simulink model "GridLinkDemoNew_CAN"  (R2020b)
settings: Solver=FixedStepDiscrete  StartTime=0.0  StopTime=inf  RelTol=1e-3  EnableMultiTasking=on
InitFcn:
  | INNER_PWM=1000
  | OUTER_PWM=50000
undefined symbols (not defined in the file): A, ADCIN0, ADCIN1, ADCINA0, ADCINB0, bit, Compare, conversion, CounterCut_Outer, DCAEVT1, DCAEVT1FILT, Digital, Down, ended, Event, Filtered, GPTRIP1SEL, GPTRIP2SEL, hex2dec, identifier, input, Module, Newinv, of, Single, SPS_EMT_TAPAS_2018b, Standard, start, Tmod1, Trip, TZ1, TZ2, U_dc, Up, version, Zone
libraries: tiiqmathlib x63, c2802xlib x31, c2837xDlib x5, c280xlib x5, c28xdmclib x2, simulink x2, svdutilitieslib x1, c2000lib x1, canmsglib x1
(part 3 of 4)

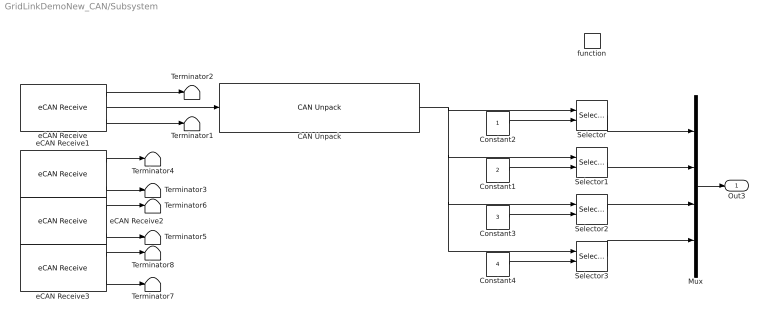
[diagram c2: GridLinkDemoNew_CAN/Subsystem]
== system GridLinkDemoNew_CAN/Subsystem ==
  function : TriggerPort  TriggerType=function-call  VariantControl=Variant
  CAN Unpack : canmsglib/CAN Unpack  MsgList=(none)  MsgName=CAN Msg  MsgIDType=Standard (11-bit identifier)  MsgIdentifier=hex2dec('01A')  MsgLength=4  SignalInfo={}  IDPort=off  TimestampPort=off  ErrorPort=off  RemotePort=off  LengthPort=off  StatusPort=off  ApplyMinMax=off
  Constant1 : Constant  Value=2  OutDataTypeStr=Inherit: Inherit via back propagation
  Constant2 : Constant  OutDataTypeStr=Inherit: Inherit via back propagation
  Constant3 : Constant  Value=3  OutDataTypeStr=Inherit: Inherit via back propagation
  Constant4 : Constant  Value=4  OutDataTypeStr=Inherit: Inherit via back propagation
  Mux : Mux
  Selector{,1..3} (4 alike) : Selector  InputPortWidth=4  IndexOptions=Index vector (port)  Indices=1  OutputSizes=1
  Terminator{1..8} (8 alike) : Terminator
  eCAN Receive : c280xlib/eCAN Receive  chipFamily=C280x  useModule=eCAN_B  mailboxNo=2  messageID=hex2dec('01A')  messageType=Standard (11-bit identifier)  sampleTime=-1  dataType=CAN_MESSAGE_TYPE  initValue=0  outputMessageLength=on  outputMessageTimeStamp=off  postInterrupt=on  interruptLine=0
  eCAN Receive1 : c280xlib/eCAN Receive  Commented=on  chipFamily=C280x  useModule=eCAN_B  mailboxNo=3  messageID=hex2dec('02A')  messageType=Standard (11-bit identifier)  sampleTime=-1  dataType=uint16  initValue=0  outputMessageLength=on  outputMessageTimeStamp=off  postInterrupt=on  interruptLine=0
  eCAN Receive2 : c280xlib/eCAN Receive  Commented=on  chipFamily=C280x  useModule=eCAN_B  mailboxNo=4  messageID=hex2dec('03A')  messageType=Standard (11-bit identifier)  sampleTime=-1  dataType=uint16  initValue=0  outputMessageLength=on  outputMessageTimeStamp=off  postInterrupt=on  interruptLine=0
  eCAN Receive3 : c280xlib/eCAN Receive  Commented=on  chipFamily=C280x  useModule=eCAN_B  mailboxNo=5  messageID=hex2dec('04A')  messageType=Standard (11-bit identifier)  sampleTime=-1  dataType=uint16  initValue=0  outputMessageLength=on  outputMessageTimeStamp=off  postInterrupt=on  interruptLine=0
  Out3 : Outport  VectorParamsAs1DForOutWhenUnconnected=off
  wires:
  eCAN Receive/1 -> Terminator2/1
  Constant2/1 -> Selector/2
  eCAN Receive/3 -> Terminator1/1
  eCAN Receive1/3 -> Terminator3/1
  Constant1/1 -> Selector1/2
  Selector1/1 -> Mux/2
  eCAN Receive1/1 -> Terminator4/1
  Constant3/1 -> Selector2/2
  eCAN Receive2/3 -> Terminator5/1
  Selector2/1 -> Mux/3
  eCAN Receive2/1 -> Terminator6/1
  Constant4/1 -> Selector3/2
  eCAN Receive3/3 -> Terminator7/1
  Selector3/1 -> Mux/4
  eCAN Receive3/1 -> Terminator8/1
  Mux/1 -> Out3/1
  Selector/1 -> Mux/1
  CAN Unpack/1 -> Selector3/1, Selector2/1, Selector1/1, Selector/1
  eCAN Receive/2 -> CAN Unpack/1

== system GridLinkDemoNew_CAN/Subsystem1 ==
  ePWM : c2802xlib/ePWM  PwmType=C2000_Type4  useModule=ePWM8  ePWMxLINKTBPRD=Not Linked  periodUnits=Clock cycles  timerSource=Specify via dialog  timerPeriod_clk=250  timerPeriod_sec=0.0001  tbshadow=Counter equals to zero  countingMode=Up-Down  phaseActiveEnable=Disable  phaseDirection=Count down after sync  phaseActive=0  synchronizationEnable=off  dcaevt1Sync=off  dcbevt1Sync=off  synchronizationOption=Disable  perSynchronizationOption=Counter equals to period (CTR=PRD)  clockPrescale=1  HSclockPrescale=1  enswap=off  ePWMxAStatus=on  ePWMxAactionLogic1=Do nothing  ePWMxAactionLogic2=Do nothing  ePWMxAactionLogic3=Set  ePWMxAactionLogic4=Clear  ePWMxAactionLogic5=Do nothing  ePWMxAactionLogic6=Do nothing  ePWMxACSFenable=off  ePWMxACSFvalue=Forcing disable  ePWMxASFreload=Zero  ePWMxBStatus=on  ePWMxBactionLogic1=Do nothing  ePWMxBactionLogic2=Do nothing  ePWMxBactionLogic3=Do nothing  ePWMxBactionLogic4=Do nothing  ePWMxBactionLogic5=Do nothing  ePWMxBactionLogic6=Do nothing  ePWMxBCSFenable=off  ePWMxBCSFvalue=Forcing disable  ePWMxBSFreload=Zero  ePWNxBOutWay=off  ePWMxLINKCMPA=Not Linked  CMPAUnits=Clock cycles  CMPASource=Specify via dialog  CMPAValue_per=50  CMPAValue_clk=10  enCMPAshadow=Counter equals to zero (CTR=Zero)  ePWMxLINKCMPB=Not Linked  CMPBUnits=Clock cycles  CMPBSource=Specify via dialog  CMPBValue_per=50  CMPBValue_clk=0  enCMPBshadow=Counter equals to zero (CTR=Zero)  ePWMxLINKCMPC=Not Linked  CMPCUnits=Clock cycles  CMPCSource=Specify via dialog  CMPCValue_per=50  CMPCValue_clk=0  enCMPCshadow=Counter equals to zero (CTR=Zero)  ePWMxLINKCMPD=Not Linked  CMPDUnits=Clock cycles  CMPDSource=Specify via dialog  CMPDValue_per=50  CMPDValue_clk=0  enCMPDshadow=Counter equals to zero (CTR=Zero)  enableDBePWMxA=off  enableDBePWMxB=off  enhalfcycle=off  DBpolarity=Active high (AH)  DBedgeDelay=Positive  DBSource_ePWMxA=ePWMxA  DBSource_ePWMxB=ePWMxA  DBPeriodUnits=Clock cycles  DBperiodSource=Specify via dialog  REDperiod=0  FEDperiod=0  REDperiod_sec=0  FEDperiod_sec=0  LoadModeDBRED=Immediate without using shadow  LoadModeDBFED=Immediate without using shadow  adcstartModuleA=off  adcrequestEventA=First event  adcstartEventA=Digital Compare Module A Event 1 start of conversion (DCAEVT1.soc)  adcstartEventA_type2=Counter equals to period (CTR=PRD)  adcstartModuleB=off  adcrequestEventB=First event  adcstartEventB=Counter equals to zero (CTR=Zero)  adcstartEventB_type2=Counter equals to zero (CTR=Zero)  intEn=on  intPrd=Third event  intSel=Counter equals to zero (CTR=Zero)  intSel_type2=Counter equals to zero (CTR=Zero)  hrpe=off  enHRPWM=off  HRPWM_LoadMode=Counter equals to period (CTR=PRD)  HRPWM_CTLMode=Duty or Period control mode  HRPWM_EDGMode=Both edge  hrpeb=off  enHRPWMB=off  HRPWM_LoadModeB=Counter equals to zero (CTR=ZERO)  HRPWM_CTLModeB=Duty or Period control mode  HRPWM_EDGModeB=Both edge  enHRDBRED=off  enHRDBFED=off  enSFO=on  enautoconv=on  chopperEnable=off  chopperFrequency=1  chopperFirstwidth=1  chopperDuty=12.5%  tripZonesource=Specify via dialog  tzselOSHT1=off  tzselOSHT2=off  tzselOSHT3=off  tzselOSHDCAEV1=off  tzselOSHDCBEV1=off  tzselCBC1=off  tzselCBC2=off  tzselCBC3=off  tzselCBCDCAEV2=off  tzselCBCDCBEV2=off  tzselOSHT4=off  tzselOSHT5=off  tzselOSHT6=off  tzselCBC4=off  tzselCBC5=off  tzselCBC6=off  enTzOstIntr=off  enTzCbcIntr=off  enTzDCAEVT1Intr=off  enTzDCAEVT2Intr=off  enTzDCBEVT1Intr=off  enTzDCBEVT2Intr=off  ePWMxAforced=No action  ePWMxBforced=No action  DCAEVT1forced=No action  DCBEVT1forced=No action  DCAEVT2forced=No action  DCBEVT2forced=No action  dcah=Trip Zone 1 input (TZ1)  dcal=Trip Zone 2 input (TZ2)  dcbh=Trip Zone 1 input (TZ1)  dcbl=Trip Zone 2 input (TZ2)  dcah_type2=GPTRIP1SEL/(TZ1)  dcal_type2=GPTRIP2SEL/(TZ2)  dcbh_type2=GPTRIP1SEL/(TZ1)  dcbl_type2=GPTRIP2SEL/(TZ2)  gendcaevt1=Event disabled  gendcaevt2=Event disabled  gendcbevt1=Event disabled  gendcbevt2=Event disabled  dcaevt1src=DCAEVT1 with sync  dcaevt2src=DCAEVT2 with sync  dcbevt1src=DCBEVT1 with sync  dcbevt2src=DCBEVT2 with sync  pulsesel=Counter equals to zero (CTR=Zero)  blankinv=off  blankoffset=0  blankwidth=0  evsrcsel=Filtered version of DCAEVT1 (DCAEVT1FILT)  encape=off

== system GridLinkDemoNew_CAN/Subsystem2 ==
  note: counter +=
  note: Reset counter
  function : TriggerPort  TriggerType=function-call  VariantControl=Variant
  Data Store Read1 : DataStoreRead  DataStoreName=CounterCut
  Data Store Read2 : DataStoreRead  DataStoreName=Counter
  If : If  NumInputs=2  IfExpression=u1 >= u2
  If Action Subsystem : Subsystem  TreatAsAtomicUnit=on
  If Action Subsystem1 : Subsystem  TreatAsAtomicUnit=on
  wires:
  Data Store Read2/1 -> If/1
  Data Store Read1/1 -> If/2
  If/2 -> If Action Subsystem1/Action
  If/1 -> If Action Subsystem/Action

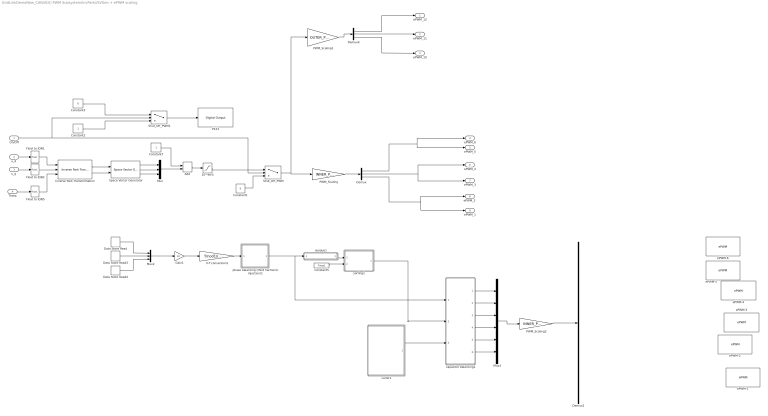
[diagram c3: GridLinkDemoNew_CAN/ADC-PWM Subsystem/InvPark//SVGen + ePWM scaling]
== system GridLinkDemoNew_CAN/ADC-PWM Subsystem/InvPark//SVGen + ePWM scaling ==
  On/Off : Inport
  "u_d " : Inport  Port=2
  "u_q " : Inport  Port=3
  Theta : Inport  Port=4
  10~90% : Saturate  UpperLimit=1.8  LowerLimit=0.2  OutDataTypeStr=Inherit: Inherit via back propagation
  Add : Sum
  Constant1 : Constant  Value=0  OutDataTypeStr=Inherit: Inherit via back propagation
  Constant2 : Constant  OutDataTypeStr=boolean
  Constant3 : Constant  Value=0  OutDataTypeStr=boolean
  Constant5 : Constant  Commented=on  Value=Tmod1  OutDataTypeStr=single
  Constant7 : Constant  OutDataTypeStr=Inherit: Inherit via back propagation
  Data Store Read : DataStoreRead  Commented=on  DataStoreName=Ua
  Data Store Read3 : DataStoreRead  Commented=on  DataStoreName=Ub
  Data Store Read4 : DataStoreRead  Commented=on  DataStoreName=Uc
  Demux : Demux  Outputs=3
  Demux2 : Demux  Commented=on  Outputs=6
  Demux4 : Demux  Outputs=3
  Float to IQN1 : tiiqmathlib/Float to IQN  Q_value=16
  Float to IQN2 : tiiqmathlib/Float to IQN  Q_value=16
  Float to IQN5 : tiiqmathlib/Float to IQN  Q_value=16
  Gain1 : Gain  Commented=on  Gain=10  OutDataTypeStr=single
  Inverse Park Transformation : c28xdmclib/Inverse Park Transformation
  Mux : Mux  Inputs=3
  Mux2 : Mux  Commented=on  Inputs=3
  Mux3 : Mux  Commented=on  Inputs=6
  P123 : c2837xDlib/Digital Output  GPIO_Number=GPIO112~GPIO119  GPIO_Bit0=off  GPIO_BIT0_Toggle=on  GPIO_Bit1=off  GPIO_BIT1_Toggle=on  GPIO_Bit2=off  GPIO_BIT2_Toggle=off  GPIO_Bit3=off  GPIO_BIT3_Toggle=off  GPIO_Bit4=off  GPIO_BIT4_Toggle=off  GPIO_Bit5=off  GPIO_BIT5_Toggle=on  GPIO_Bit6=off  GPIO_BIT6_Toggle=off  GPIO_Bit7=on  GPIO_BIT7_Toggle=off
  PWM_Scaling : Gain  Gain=INNER_PWM/2  ParamDataTypeStr=Inherit: Inherit from 'Gain'  OutDataTypeStr=Inherit: Inherit via back propagation
  PWM_Scaling1 : Gain  Gain=OUTER_PWM/2  ParamDataTypeStr=Inherit: Inherit from 'Gain'  OutDataTypeStr=Inherit: Inherit via back propagation
  PWM_Scaling2 : Gain  Commented=on  Gain=INNER_PWM/2  ParamDataTypeStr=Inherit: Inherit from 'Gain'  OutDataTypeStr=Inherit: Inherit via back propagation
  Shut_Off_PWM : Switch  Criteria=u2 > Threshold  OutDataTypeStr=Inherit: Inherit via back propagation
  Shut_Off_PWM1 : Switch  Criteria=u2 > Threshold  OutDataTypeStr=Inherit: Inherit via back propagation
  Space Vector Generator : c28xdmclib/Space Vector Generator
  V-T conversion1 : Gain  Commented=on  Gain=Tmod1/(U_dc/2)  OutDataTypeStr=single  SaturateOnIntegerOverflow=on
  capacitor balancing1 : Subsystem  Commented=on
  carier1 : Subsystem  Commented=on
  "ePWM-1 " : c2802xlib/ePWM  Commented=on  PwmType=C2000_Type4  useModule=ePWM1  ePWMxLINKTBPRD=Not Linked  periodUnits=Clock cycles  timerSource=Specify via dialog  timerPeriod_clk=INNER_PWM  timerPeriod_sec=0.0001  tbshadow=Counter equals to zero  countingMode=Up-Down  phaseActiveEnable=Set counter to phase value specified via dialog  phaseDirection=Count down after sync  phaseActive=0  synchronizationEnable=off  dcaevt1Sync=off  dcbevt1Sync=off  synchronizationOption=Disable  perSynchronizationOption=Counter equals to period (CTR=PRD)  clockPrescale=1  HSclockPrescale=1  enswap=off  ePWMxAStatus=on  ePWMxAactionLogic1=Do nothing  ePWMxAactionLogic2=Do nothing  ePWMxAactionLogic3=Clear  ePWMxAactionLogic4=Set  ePWMxAactionLogic5=Do nothing  ePWMxAactionLogic6=Do nothing  ePWMxACSFenable=off  ePWMxACSFvalue=Forcing disable  ePWMxASFreload=Immediate  ePWMxBStatus=off  ePWMxBactionLogic1=Do nothing  ePWMxBactionLogic2=Do nothing  ePWMxBactionLogic3=Clear  ePWMxBactionLogic4=Set  ePWMxBactionLogic5=Do nothing  ePWMxBactionLogic6=Do nothing  ePWMxBCSFenable=off  ePWMxBCSFvalue=Forcing disable  ePWMxBSFreload=Immediate  ePWNxBOutWay=off  ePWMxLINKCMPA=Not Linked  CMPAUnits=Clock cycles  CMPASource=Input port  CMPAValue_per=50  CMPAValue_clk=0  enCMPAshadow=Counter equals to zero (CTR=Zero)  ePWMxLINKCMPB=Not Linked  CMPBUnits=Clock cycles  CMPBSource=Specify via dialog  CMPBValue_per=50  CMPBValue_clk=32000  enCMPBshadow=Counter equals to zero (CTR=Zero)  ePWMxLINKCMPC=Not Linked  CMPCUnits=Clock cycles  CMPCSource=Specify via dialog  CMPCValue_per=50  CMPCValue_clk=32000  enCMPCshadow=Counter equals to zero (CTR=Zero)  ePWMxLINKCMPD=Not Linked  CMPDUnits=Clock cycles  CMPDSource=Specify via dialog  CMPDValue_per=50  CMPDValue_clk=32000  enCMPDshadow=Counter equals to zero (CTR=Zero)  enableDBePWMxA=on  enableDBePWMxB=on  enhalfcycle=off  DBpolarity=Active high complementary (AHC)  DBedgeDelay=Positive  DBSource_ePWMxA=ePWMxA  DBSource_ePWMxB=ePWMxA  DBPeriodUnits=Clock cycles  DBperiodSource=Specify via dialog  REDperiod=2  FEDperiod=2  REDperiod_sec=0  FEDperiod_sec=0  LoadModeDBRED=Immediate without using shadow  LoadModeDBFED=Immediate without using shadow  adcstartModuleA=off  adcrequestEventA=First event  adcstartEventA=Digital Compare Module A Event 1 start of conversion (DCAEVT1.soc)  adcstartEventA_type2=Counter equals to period (CTR=PRD)  adcstartModuleB=off  adcrequestEventB=First event  adcstartEventB=Counter equals to zero (CTR=Zero)  adcstartEventB_type2=Counter equals to zero (CTR=Zero)  intEn=off  intPrd=First event  intSel=Counter equals to zero (CTR=Zero)  intSel_type2=Counter equals to zero (CTR=Zero)  hrpe=off  enHRPWM=off  HRPWM_LoadMode=Counter equals to period (CTR=PRD)  HRPWM_CTLMode=Duty or Period control mode  HRPWM_EDGMode=Both edge  hrpeb=off  enHRPWMB=off  HRPWM_LoadModeB=Counter equals to zero (CTR=ZERO)  HRPWM_CTLModeB=Duty or Period control mode  HRPWM_EDGModeB=Both edge  enHRDBRED=off  enHRDBFED=off  enSFO=on  enautoconv=on  chopperEnable=off  chopperFrequency=1  chopperFirstwidth=1  chopperDuty=12.5%  tripZonesource=Specify via dialog  tzselOSHT1=off  tzselOSHT2=off  tzselOSHT3=off  tzselOSHDCAEV1=off  tzselOSHDCBEV1=off  tzselCBC1=off  tzselCBC2=off  tzselCBC3=off  tzselCBCDCAEV2=off  tzselCBCDCBEV2=off  tzselOSHT4=off  tzselOSHT5=off  tzselOSHT6=off  tzselCBC4=off  tzselCBC5=off  tzselCBC6=off  enTzOstIntr=off  enTzCbcIntr=off  enTzDCAEVT1Intr=off  enTzDCAEVT2Intr=off  enTzDCBEVT1Intr=off  enTzDCBEVT2Intr=off  ePWMxAforced=No action  ePWMxBforced=No action  DCAEVT1forced=No action  DCBEVT1forced=No action  DCAEVT2forced=No action  DCBEVT2forced=No action  dcah=Trip Zone 1 input (TZ1)  dcal=Trip Zone 2 input (TZ2)  dcbh=Trip Zone 1 input (TZ1)  dcbl=Trip Zone 2 input (TZ2)  dcah_type2=GPTRIP1SEL/(TZ1)  dcal_type2=GPTRIP2SEL/(TZ2)  dcbh_type2=GPTRIP1SEL/(TZ1)  dcbl_type2=GPTRIP2SEL/(TZ2)  gendcaevt1=Event disabled  gendcaevt2=Event disabled  gendcbevt1=Event disabled  gendcbevt2=Event disabled  dcaevt1src=DCAEVT1 with sync  dcaevt2src=DCAEVT2 with sync  dcbevt1src=DCBEVT1 with sync  dcbevt2src=DCBEVT2 with sync  pulsesel=Counter equals to zero (CTR=Zero)  blankinv=off  blankoffset=0  blankwidth=0  evsrcsel=Filtered version of DCAEVT1 (DCAEVT1FILT)  encape=off
  "ePWM-2 " : c2802xlib/ePWM  Commented=on  PwmType=C2000_Type4  useModule=ePWM2  ePWMxLINKTBPRD=Not Linked  periodUnits=Clock cycles  timerSource=Specify via dialog  timerPeriod_clk=INNER_PWM  timerPeriod_sec=0.0001  tbshadow=Counter equals to zero  countingMode=Up-Down  phaseActiveEnable=Set counter to phase value specified via dialog  phaseDirection=Count down after sync  phaseActive=0  synchronizationEnable=off  dcaevt1Sync=off  dcbevt1Sync=off  synchronizationOption=Disable  perSynchronizationOption=Counter equals to period (CTR=PRD)  clockPrescale=1  HSclockPrescale=1  enswap=off  ePWMxAStatus=on  ePWMxAactionLogic1=Do nothing  ePWMxAactionLogic2=Do nothing  ePWMxAactionLogic3=Clear  ePWMxAactionLogic4=Set  ePWMxAactionLogic5=Do nothing  ePWMxAactionLogic6=Do nothing  ePWMxACSFenable=off  ePWMxACSFvalue=Forcing disable  ePWMxASFreload=Immediate  ePWMxBStatus=off  ePWMxBactionLogic1=Do nothing  ePWMxBactionLogic2=Do nothing  ePWMxBactionLogic3=Clear  ePWMxBactionLogic4=Set  ePWMxBactionLogic5=Do nothing  ePWMxBactionLogic6=Do nothing  ePWMxBCSFenable=off  ePWMxBCSFvalue=Forcing disable  ePWMxBSFreload=Immediate  ePWNxBOutWay=off  ePWMxLINKCMPA=Not Linked  CMPAUnits=Clock cycles  CMPASource=Input port  CMPAValue_per=50  CMPAValue_clk=0  enCMPAshadow=Counter equals to zero (CTR=Zero)  ePWMxLINKCMPB=Not Linked  CMPBUnits=Clock cycles  CMPBSource=Specify via dialog  CMPBValue_per=50  CMPBValue_clk=32000  enCMPBshadow=Counter equals to zero (CTR=Zero)  ePWMxLINKCMPC=Not Linked  CMPCUnits=Clock cycles  CMPCSource=Specify via dialog  CMPCValue_per=50  CMPCValue_clk=32000  enCMPCshadow=Counter equals to zero (CTR=Zero)  ePWMxLINKCMPD=Not Linked  CMPDUnits=Clock cycles  CMPDSource=Specify via dialog  CMPDValue_per=50  CMPDValue_clk=32000  enCMPDshadow=Counter equals to zero (CTR=Zero)  enableDBePWMxA=on  enableDBePWMxB=on  enhalfcycle=off  DBpolarity=Active high complementary (AHC)  DBedgeDelay=Positive  DBSource_ePWMxA=ePWMxA  DBSource_ePWMxB=ePWMxA  DBPeriodUnits=Clock cycles  DBperiodSource=Specify via dialog  REDperiod=2  FEDperiod=2  REDperiod_sec=0  FEDperiod_sec=0  LoadModeDBRED=Immediate without using shadow  LoadModeDBFED=Immediate without using shadow  adcstartModuleA=off  adcrequestEventA=First event  adcstartEventA=Digital Compare Module A Event 1 start of conversion (DCAEVT1.soc)  adcstartEventA_type2=Counter equals to period (CTR=PRD)  adcstartModuleB=off  adcrequestEventB=First event  adcstartEventB=Counter equals to zero (CTR=Zero)  adcstartEventB_type2=Counter equals to zero (CTR=Zero)  intEn=off  intPrd=First event  intSel=Counter equals to zero (CTR=Zero)  intSel_type2=Counter equals to zero (CTR=Zero)  hrpe=off  enHRPWM=off  HRPWM_LoadMode=Counter equals to period (CTR=PRD)  HRPWM_CTLMode=Duty or Period control mode  HRPWM_EDGMode=Both edge  hrpeb=off  enHRPWMB=off  HRPWM_LoadModeB=Counter equals to zero (CTR=ZERO)  HRPWM_CTLModeB=Duty or Period control mode  HRPWM_EDGModeB=Both edge  enHRDBRED=off  enHRDBFED=off  enSFO=on  enautoconv=on  chopperEnable=off  chopperFrequency=1  chopperFirstwidth=1  chopperDuty=12.5%  tripZonesource=Specify via dialog  tzselOSHT1=off  tzselOSHT2=off  tzselOSHT3=off  tzselOSHDCAEV1=off  tzselOSHDCBEV1=off  tzselCBC1=off  tzselCBC2=off  tzselCBC3=off  tzselCBCDCAEV2=off  tzselCBCDCBEV2=off  tzselOSHT4=off  tzselOSHT5=off  tzselOSHT6=off  tzselCBC4=off  tzselCBC5=off  tzselCBC6=off  enTzOstIntr=off  enTzCbcIntr=off  enTzDCAEVT1Intr=off  enTzDCAEVT2Intr=off  enTzDCBEVT1Intr=off  enTzDCBEVT2Intr=off  ePWMxAforced=No action  ePWMxBforced=No action  DCAEVT1forced=No action  DCBEVT1forced=No action  DCAEVT2forced=No action  DCBEVT2forced=No action  dcah=Trip Zone 1 input (TZ1)  dcal=Trip Zone 2 input (TZ2)  dcbh=Trip Zone 1 input (TZ1)  dcbl=Trip Zone 2 input (TZ2)  dcah_type2=GPTRIP1SEL/(TZ1)  dcal_type2=GPTRIP2SEL/(TZ2)  dcbh_type2=GPTRIP1SEL/(TZ1)  dcbl_type2=GPTRIP2SEL/(TZ2)  gendcaevt1=Event disabled  gendcaevt2=Event disabled  gendcbevt1=Event disabled  gendcbevt2=Event disabled  dcaevt1src=DCAEVT1 with sync  dcaevt2src=DCAEVT2 with sync  dcbevt1src=DCBEVT1 with sync  dcbevt2src=DCBEVT2 with sync  pulsesel=Counter equals to zero (CTR=Zero)  blankinv=off  blankoffset=0  blankwidth=0  evsrcsel=Filtered version of DCAEVT1 (DCAEVT1FILT)  encape=off
  ePWM-3 : c2802xlib/ePWM  Commented=on  PwmType=C2000_Type4  useModule=ePWM3  ePWMxLINKTBPRD=Not Linked  periodUnits=Clock cycles  timerSource=Specify via dialog  timerPeriod_clk=INNER_PWM  timerPeriod_sec=0.0001  tbshadow=Counter equals to zero  countingMode=Up-Down  phaseActiveEnable=Set counter to phase value specified via dialog  phaseDirection=Count up after sync  phaseActive=0  synchronizationEnable=off  dcaevt1Sync=off  dcbevt1Sync=off  synchronizationOption=Pass through (EPWMxSYNCI or SWFSYNC)  perSynchronizationOption=Counter equals to period (CTR=PRD)  clockPrescale=1  HSclockPrescale=1  enswap=off  ePWMxAStatus=on  ePWMxAactionLogic1=Do nothing  ePWMxAactionLogic2=Do nothing  ePWMxAactionLogic3=Clear  ePWMxAactionLogic4=Set  ePWMxAactionLogic5=Do nothing  ePWMxAactionLogic6=Do nothing  ePWMxACSFenable=off  ePWMxACSFvalue=Forcing disable  ePWMxASFreload=Immediate  ePWMxBStatus=off  ePWMxBactionLogic1=Do nothing  ePWMxBactionLogic2=Do nothing  ePWMxBactionLogic3=Clear  ePWMxBactionLogic4=Set  ePWMxBactionLogic5=Do nothing  ePWMxBactionLogic6=Do nothing  ePWMxBCSFenable=off  ePWMxBCSFvalue=Forcing disable  ePWMxBSFreload=Immediate  ePWNxBOutWay=off  ePWMxLINKCMPA=Not Linked  CMPAUnits=Clock cycles  CMPASource=Input port  CMPAValue_per=50  CMPAValue_clk=0  enCMPAshadow=Counter equals to zero (CTR=Zero)  ePWMxLINKCMPB=Not Linked  CMPBUnits=Clock cycles  CMPBSource=Specify via dialog  CMPBValue_per=50  CMPBValue_clk=32000  enCMPBshadow=Counter equals to zero (CTR=Zero)  ePWMxLINKCMPC=Not Linked  CMPCUnits=Clock cycles  CMPCSource=Specify via dialog  CMPCValue_per=50  CMPCValue_clk=32000  enCMPCshadow=Counter equals to zero (CTR=Zero)  ePWMxLINKCMPD=Not Linked  CMPDUnits=Clock cycles  CMPDSource=Specify via dialog  CMPDValue_per=50  CMPDValue_clk=32000  enCMPDshadow=Counter equals to zero (CTR=Zero)  enableDBePWMxA=on  enableDBePWMxB=on  enhalfcycle=off  DBpolarity=Active high complementary (AHC)  DBedgeDelay=Positive  DBSource_ePWMxA=ePWMxA  DBSource_ePWMxB=ePWMxA  DBPeriodUnits=Clock cycles  DBperiodSource=Specify via dialog  REDperiod=2  FEDperiod=2  REDperiod_sec=0  FEDperiod_sec=0  LoadModeDBRED=Immediate without using shadow  LoadModeDBFED=Immediate without using shadow  adcstartModuleA=off  adcrequestEventA=First event  adcstartEventA=Digital Compare Module A Event 1 start of conversion (DCAEVT1.soc)  adcstartEventA_type2=Counter equals to period (CTR=PRD)  adcstartModuleB=off  adcrequestEventB=First event  adcstartEventB=Counter equals to zero (CTR=Zero)  adcstartEventB_type2=Counter equals to zero (CTR=Zero)  intEn=off  intPrd=First event  intSel=Counter equals to zero (CTR=Zero)  intSel_type2=Counter equals to zero (CTR=Zero)  hrpe=off  enHRPWM=off  HRPWM_LoadMode=Counter equals to period (CTR=PRD)  HRPWM_CTLMode=Duty or Period control mode  HRPWM_EDGMode=Both edge  hrpeb=off  enHRPWMB=off  HRPWM_LoadModeB=Counter equals to zero (CTR=ZERO)  HRPWM_CTLModeB=Duty or Period control mode  HRPWM_EDGModeB=Both edge  enHRDBRED=off  enHRDBFED=off  enSFO=on  enautoconv=on  chopperEnable=off  chopperFrequency=1  chopperFirstwidth=1  chopperDuty=12.5%  tripZonesource=Specify via dialog  tzselOSHT1=off  tzselOSHT2=off  tzselOSHT3=off  tzselOSHDCAEV1=off  tzselOSHDCBEV1=off  tzselCBC1=off  tzselCBC2=off  tzselCBC3=off  tzselCBCDCAEV2=off  tzselCBCDCBEV2=off  tzselOSHT4=off  tzselOSHT5=off  tzselOSHT6=off  tzselCBC4=off  tzselCBC5=off  tzselCBC6=off  enTzOstIntr=off  enTzCbcIntr=off  enTzDCAEVT1Intr=off  enTzDCAEVT2Intr=off  enTzDCBEVT1Intr=off  enTzDCBEVT2Intr=off  ePWMxAforced=No action  ePWMxBforced=No action  DCAEVT1forced=No action  DCBEVT1forced=No action  DCAEVT2forced=No action  DCBEVT2forced=No action  dcah=Trip Zone 1 input (TZ1)  dcal=Trip Zone 2 input (TZ2)  dcbh=Trip Zone 1 input (TZ1)  dcbl=Trip Zone 2 input (TZ2)  dcah_type2=GPTRIP1SEL/(TZ1)  dcal_type2=GPTRIP2SEL/(TZ2)  dcbh_type2=GPTRIP1SEL/(TZ1)  dcbl_type2=GPTRIP2SEL/(TZ2)  gendcaevt1=Event disabled  gendcaevt2=Event disabled  gendcbevt1=Event disabled  gendcbevt2=Event disabled  dcaevt1src=DCAEVT1 with sync  dcaevt2src=DCAEVT2 with sync  dcbevt1src=DCBEVT1 with sync  dcbevt2src=DCBEVT2 with sync  pulsesel=Counter equals to zero (CTR=Zero)  blankinv=off  blankoffset=0  blankwidth=0  evsrcsel=Filtered version of DCAEVT1 (DCAEVT1FILT)  encape=off
  ePWM-4 : c2802xlib/ePWM  Commented=on  PwmType=C2000_Type4  useModule=ePWM4  ePWMxLINKTBPRD=Not Linked  periodUnits=Clock cycles  timerSource=Specify via dialog  timerPeriod_clk=INNER_PWM  timerPeriod_sec=0.0001  tbshadow=Counter equals to zero  countingMode=Up-Down  phaseActiveEnable=Set counter to phase value specified via dialog  phaseDirection=Count up after sync  phaseActive=0  synchronizationEnable=off  dcaevt1Sync=off  dcbevt1Sync=off  synchronizationOption=Pass through (EPWMxSYNCI or SWFSYNC)  perSynchronizationOption=Counter equals to period (CTR=PRD)  clockPrescale=1  HSclockPrescale=1  enswap=off  ePWMxAStatus=on  ePWMxAactionLogic1=Do nothing  ePWMxAactionLogic2=Do nothing  ePWMxAactionLogic3=Clear  ePWMxAactionLogic4=Set  ePWMxAactionLogic5=Do nothing  ePWMxAactionLogic6=Do nothing  ePWMxACSFenable=off  ePWMxACSFvalue=Forcing disable  ePWMxASFreload=Immediate  ePWMxBStatus=off  ePWMxBactionLogic1=Do nothing  ePWMxBactionLogic2=Do nothing  ePWMxBactionLogic3=Clear  ePWMxBactionLogic4=Set  ePWMxBactionLogic5=Do nothing  ePWMxBactionLogic6=Do nothing  ePWMxBCSFenable=off  ePWMxBCSFvalue=Forcing disable  ePWMxBSFreload=Immediate  ePWNxBOutWay=off  ePWMxLINKCMPA=Not Linked  CMPAUnits=Clock cycles  CMPASource=Input port  CMPAValue_per=50  CMPAValue_clk=0  enCMPAshadow=Counter equals to zero (CTR=Zero)  ePWMxLINKCMPB=Not Linked  CMPBUnits=Clock cycles  CMPBSource=Specify via dialog  CMPBValue_per=50  CMPBValue_clk=32000  enCMPBshadow=Counter equals to zero (CTR=Zero)  ePWMxLINKCMPC=Not Linked  CMPCUnits=Clock cycles  CMPCSource=Specify via dialog  CMPCValue_per=50  CMPCValue_clk=32000  enCMPCshadow=Counter equals to zero (CTR=Zero)  ePWMxLINKCMPD=Not Linked  CMPDUnits=Clock cycles  CMPDSource=Specify via dialog  CMPDValue_per=50  CMPDValue_clk=32000  enCMPDshadow=Counter equals to zero (CTR=Zero)  enableDBePWMxA=on  enableDBePWMxB=on  enhalfcycle=off  DBpolarity=Active high complementary (AHC)  DBedgeDelay=Positive  DBSource_ePWMxA=ePWMxA  DBSource_ePWMxB=ePWMxA  DBPeriodUnits=Clock cycles  DBperiodSource=Specify via dialog  REDperiod=2  FEDperiod=2  REDperiod_sec=0  FEDperiod_sec=0  LoadModeDBRED=Immediate without using shadow  LoadModeDBFED=Immediate without using shadow  adcstartModuleA=off  adcrequestEventA=First event  adcstartEventA=Digital Compare Module A Event 1 start of conversion (DCAEVT1.soc)  adcstartEventA_type2=Counter equals to period (CTR=PRD)  adcstartModuleB=off  adcrequestEventB=First event  adcstartEventB=Counter equals to zero (CTR=Zero)  adcstartEventB_type2=Counter equals to zero (CTR=Zero)  intEn=off  intPrd=First event  intSel=Counter equals to zero (CTR=Zero)  intSel_type2=Counter equals to zero (CTR=Zero)  hrpe=off  enHRPWM=off  HRPWM_LoadMode=Counter equals to period (CTR=PRD)  HRPWM_CTLMode=Duty or Period control mode  HRPWM_EDGMode=Both edge  hrpeb=off  enHRPWMB=off  HRPWM_LoadModeB=Counter equals to zero (CTR=ZERO)  HRPWM_CTLModeB=Duty or Period control mode  HRPWM_EDGModeB=Both edge  enHRDBRED=off  enHRDBFED=off  enSFO=on  enautoconv=on  chopperEnable=off  chopperFrequency=1  chopperFirstwidth=1  chopperDuty=12.5%  tripZonesource=Specify via dialog  tzselOSHT1=off  tzselOSHT2=off  tzselOSHT3=off  tzselOSHDCAEV1=off  tzselOSHDCBEV1=off  tzselCBC1=off  tzselCBC2=off  tzselCBC3=off  tzselCBCDCAEV2=off  tzselCBCDCBEV2=off  tzselOSHT4=off  tzselOSHT5=off  tzselOSHT6=off  tzselCBC4=off  tzselCBC5=off  tzselCBC6=off  enTzOstIntr=off  enTzCbcIntr=off  enTzDCAEVT1Intr=off  enTzDCAEVT2Intr=off  enTzDCBEVT1Intr=off  enTzDCBEVT2Intr=off  ePWMxAforced=No action  ePWMxBforced=No action  DCAEVT1forced=No action  DCBEVT1forced=No action  DCAEVT2forced=No action  DCBEVT2forced=No action  dcah=Trip Zone 1 input (TZ1)  dcal=Trip Zone 2 input (TZ2)  dcbh=Trip Zone 1 input (TZ1)  dcbl=Trip Zone 2 input (TZ2)  dcah_type2=GPTRIP1SEL/(TZ1)  dcal_type2=GPTRIP2SEL/(TZ2)  dcbh_type2=GPTRIP1SEL/(TZ1)  dcbl_type2=GPTRIP2SEL/(TZ2)  gendcaevt1=Event disabled  gendcaevt2=Event disabled  gendcbevt1=Event disabled  gendcbevt2=Event disabled  dcaevt1src=DCAEVT1 with sync  dcaevt2src=DCAEVT2 with sync  dcbevt1src=DCBEVT1 with sync  dcbevt2src=DCBEVT2 with sync  pulsesel=Counter equals to zero (CTR=Zero)  blankinv=off  blankoffset=0  blankwidth=0  evsrcsel=Filtered version of DCAEVT1 (DCAEVT1FILT)  encape=off
  ePWM-5 : c2802xlib/ePWM  Commented=on  PwmType=C2000_Type4  useModule=ePWM5  ePWMxLINKTBPRD=Not Linked  periodUnits=Clock cycles  timerSource=Specify via dialog  timerPeriod_clk=INNER_PWM  timerPeriod_sec=0.0001  tbshadow=Counter equals to zero  countingMode=Up-Down  phaseActiveEnable=Disable  phaseDirection=Count down after sync  phaseActive=0  synchronizationEnable=off  dcaevt1Sync=off  dcbevt1Sync=off  synchronizationOption=Counter equals to zero (CTR=Zero)  perSynchronizationOption=Counter equals to period (CTR=PRD)  clockPrescale=1  HSclockPrescale=1  enswap=off  ePWMxAStatus=on  ePWMxAactionLogic1=Do nothing  ePWMxAactionLogic2=Do nothing  ePWMxAactionLogic3=Clear  ePWMxAactionLogic4=Set  ePWMxAactionLogic5=Do nothing  ePWMxAactionLogic6=Do nothing  ePWMxACSFenable=off  ePWMxACSFvalue=Forcing disable  ePWMxASFreload=Immediate  ePWMxBStatus=off  ePWMxBactionLogic1=Do nothing  ePWMxBactionLogic2=Do nothing  ePWMxBactionLogic3=Clear  ePWMxBactionLogic4=Set  ePWMxBactionLogic5=Do nothing  ePWMxBactionLogic6=Do nothing  ePWMxBCSFenable=off  ePWMxBCSFvalue=Forcing disable  ePWMxBSFreload=Immediate  ePWNxBOutWay=off  ePWMxLINKCMPA=Not Linked  CMPAUnits=Clock cycles  CMPASource=Input port  CMPAValue_per=50  CMPAValue_clk=0  enCMPAshadow=Counter equals to zero (CTR=Zero)  ePWMxLINKCMPB=Not Linked  CMPBUnits=Clock cycles  CMPBSource=Specify via dialog  CMPBValue_per=50  CMPBValue_clk=32000  enCMPBshadow=Counter equals to zero (CTR=Zero)  ePWMxLINKCMPC=Not Linked  CMPCUnits=Clock cycles  CMPCSource=Specify via dialog  CMPCValue_per=50  CMPCValue_clk=32000  enCMPCshadow=Counter equals to zero (CTR=Zero)  ePWMxLINKCMPD=Not Linked  CMPDUnits=Clock cycles  CMPDSource=Specify via dialog  CMPDValue_per=50  CMPDValue_clk=32000  enCMPDshadow=Counter equals to zero (CTR=Zero)  enableDBePWMxA=on  enableDBePWMxB=on  enhalfcycle=on  DBpolarity=Active high complementary (AHC)  DBedgeDelay=Positive  DBSource_ePWMxA=ePWMxA  DBSource_ePWMxB=ePWMxA  DBPeriodUnits=Clock cycles  DBperiodSource=Specify via dialog  REDperiod=2  FEDperiod=2  REDperiod_sec=0  FEDperiod_sec=0  LoadModeDBRED=Immediate without using shadow  LoadModeDBFED=Immediate without using shadow  adcstartModuleA=off  adcrequestEventA=First event  adcstartEventA=Digital Compare Module A Event 1 start of conversion (DCAEVT1.soc)  adcstartEventA_type2=Counter equals to period (CTR=PRD)  adcstartModuleB=off  adcrequestEventB=First event  adcstartEventB=Counter equals to zero (CTR=Zero)  adcstartEventB_type2=Counter equals to zero (CTR=Zero)  intEn=off  intPrd=First event  intSel=Counter equals to zero (CTR=Zero)  intSel_type2=Counter equals to zero (CTR=Zero)  hrpe=off  enHRPWM=off  HRPWM_LoadMode=Counter equals to period (CTR=PRD)  HRPWM_CTLMode=Duty or Period control mode  HRPWM_EDGMode=Both edge  hrpeb=off  enHRPWMB=off  HRPWM_LoadModeB=Counter equals to zero (CTR=ZERO)  HRPWM_CTLModeB=Duty or Period control mode  HRPWM_EDGModeB=Both edge  enHRDBRED=off  enHRDBFED=off  enSFO=on  enautoconv=on  chopperEnable=off  chopperFrequency=1  chopperFirstwidth=1  chopperDuty=12.5%  tripZonesource=Specify via dialog  tzselOSHT1=off  tzselOSHT2=off  tzselOSHT3=off  tzselOSHDCAEV1=off  tzselOSHDCBEV1=off  tzselCBC1=off  tzselCBC2=off  tzselCBC3=off  tzselCBCDCAEV2=off  tzselCBCDCBEV2=off  tzselOSHT4=off  tzselOSHT5=off  tzselOSHT6=off  tzselCBC4=off  tzselCBC5=off  tzselCBC6=off  enTzOstIntr=off  enTzCbcIntr=off  enTzDCAEVT1Intr=off  enTzDCAEVT2Intr=off  enTzDCBEVT1Intr=off  enTzDCBEVT2Intr=off  ePWMxAforced=No action  ePWMxBforced=No action  DCAEVT1forced=No action  DCBEVT1forced=No action  DCAEVT2forced=No action  DCBEVT2forced=No action  dcah=Trip Zone 1 input (TZ1)  dcal=Trip Zone 2 input (TZ2)  dcbh=Trip Zone 1 input (TZ1)  dcbl=Trip Zone 2 input (TZ2)  dcah_type2=GPTRIP1SEL/(TZ1)  dcal_type2=GPTRIP2SEL/(TZ2)  dcbh_type2=GPTRIP1SEL/(TZ1)  dcbl_type2=GPTRIP2SEL/(TZ2)  gendcaevt1=Event disabled  gendcaevt2=Event disabled  gendcbevt1=Event disabled  gendcbevt2=Event disabled  dcaevt1src=DCAEVT1 with sync  dcaevt2src=DCAEVT2 with sync  dcbevt1src=DCBEVT1 with sync  dcbevt2src=DCBEVT2 with sync  pulsesel=Counter equals to zero (CTR=Zero)  blankinv=off  blankoffset=0  blankwidth=0  evsrcsel=Filtered version of DCAEVT1 (DCAEVT1FILT)  encape=off
  ePWM-6 : c2802xlib/ePWM  Commented=on  PwmType=C2000_Type4  useModule=ePWM6  ePWMxLINKTBPRD=Not Linked  periodUnits=Clock cycles  timerSource=Specify via dialog  timerPeriod_clk=INNER_PWM  timerPeriod_sec=0.0001  tbshadow=Counter equals to zero  countingMode=Up-Down  phaseActiveEnable=Disable  phaseDirection=Count down after sync  phaseActive=0  synchronizationEnable=off  dcaevt1Sync=off  dcbevt1Sync=off  synchronizationOption=Counter equals to zero (CTR=Zero)  perSynchronizationOption=Counter equals to period (CTR=PRD)  clockPrescale=1  HSclockPrescale=1  enswap=off  ePWMxAStatus=on  ePWMxAactionLogic1=Do nothing  ePWMxAactionLogic2=Do nothing  ePWMxAactionLogic3=Clear  ePWMxAactionLogic4=Set  ePWMxAactionLogic5=Do nothing  ePWMxAactionLogic6=Do nothing  ePWMxACSFenable=off  ePWMxACSFvalue=Forcing disable  ePWMxASFreload=Immediate  ePWMxBStatus=off  ePWMxBactionLogic1=Do nothing  ePWMxBactionLogic2=Do nothing  ePWMxBactionLogic3=Clear  ePWMxBactionLogic4=Set  ePWMxBactionLogic5=Do nothing  ePWMxBactionLogic6=Do nothing  ePWMxBCSFenable=off  ePWMxBCSFvalue=Forcing disable  ePWMxBSFreload=Immediate  ePWNxBOutWay=off  ePWMxLINKCMPA=Not Linked  CMPAUnits=Clock cycles  CMPASource=Input port  CMPAValue_per=50  CMPAValue_clk=0  enCMPAshadow=Counter equals to zero (CTR=Zero)  ePWMxLINKCMPB=Not Linked  CMPBUnits=Clock cycles  CMPBSource=Specify via dialog  CMPBValue_per=50  CMPBValue_clk=32000  enCMPBshadow=Counter equals to zero (CTR=Zero)  ePWMxLINKCMPC=Not Linked  CMPCUnits=Clock cycles  CMPCSource=Specify via dialog  CMPCValue_per=50  CMPCValue_clk=32000  enCMPCshadow=Counter equals to zero (CTR=Zero)  ePWMxLINKCMPD=Not Linked  CMPDUnits=Clock cycles  CMPDSource=Specify via dialog  CMPDValue_per=50  CMPDValue_clk=32000  enCMPDshadow=Counter equals to zero (CTR=Zero)  enableDBePWMxA=on  enableDBePWMxB=on  enhalfcycle=on  DBpolarity=Active high complementary (AHC)  DBedgeDelay=Positive  DBSource_ePWMxA=ePWMxA  DBSource_ePWMxB=ePWMxA  DBPeriodUnits=Clock cycles  DBperiodSource=Specify via dialog  REDperiod=2  FEDperiod=2  REDperiod_sec=0  FEDperiod_sec=0  LoadModeDBRED=Immediate without using shadow  LoadModeDBFED=Immediate without using shadow  adcstartModuleA=off  adcrequestEventA=First event  adcstartEventA=Digital Compare Module A Event 1 start of conversion (DCAEVT1.soc)  adcstartEventA_type2=Counter equals to period (CTR=PRD)  adcstartModuleB=off  adcrequestEventB=First event  adcstartEventB=Counter equals to zero (CTR=Zero)  adcstartEventB_type2=Counter equals to zero (CTR=Zero)  intEn=off  intPrd=First event  intSel=Counter equals to zero (CTR=Zero)  intSel_type2=Counter equals to zero (CTR=Zero)  hrpe=off  enHRPWM=off  HRPWM_LoadMode=Counter equals to period (CTR=PRD)  HRPWM_CTLMode=Duty or Period control mode  HRPWM_EDGMode=Both edge  hrpeb=off  enHRPWMB=off  HRPWM_LoadModeB=Counter equals to zero (CTR=ZERO)  HRPWM_CTLModeB=Duty or Period control mode  HRPWM_EDGModeB=Both edge  enHRDBRED=off  enHRDBFED=off  enSFO=on  enautoconv=on  chopperEnable=off  chopperFrequency=1  chopperFirstwidth=1  chopperDuty=12.5%  tripZonesource=Specify via dialog  tzselOSHT1=off  tzselOSHT2=off  tzselOSHT3=off  tzselOSHDCAEV1=off  tzselOSHDCBEV1=off  tzselCBC1=off  tzselCBC2=off  tzselCBC3=off  tzselCBCDCAEV2=off  tzselCBCDCBEV2=off  tzselOSHT4=off  tzselOSHT5=off  tzselOSHT6=off  tzselCBC4=off  tzselCBC5=off  tzselCBC6=off  enTzOstIntr=off  enTzCbcIntr=off  enTzDCAEVT1Intr=off  enTzDCAEVT2Intr=off  enTzDCBEVT1Intr=off  enTzDCBEVT2Intr=off  ePWMxAforced=No action  ePWMxBforced=No action  DCAEVT1forced=No action  DCBEVT1forced=No action  DCAEVT2forced=No action  DCBEVT2forced=No action  dcah=Trip Zone 1 input (TZ1)  dcal=Trip Zone 2 input (TZ2)  dcbh=Trip Zone 1 input (TZ1)  dcbl=Trip Zone 2 input (TZ2)  dcah_type2=GPTRIP1SEL/(TZ1)  dcal_type2=GPTRIP2SEL/(TZ2)  dcbh_type2=GPTRIP1SEL/(TZ1)  dcbl_type2=GPTRIP2SEL/(TZ2)  gendcaevt1=Event disabled  gendcaevt2=Event disabled  gendcbevt1=Event disabled  gendcbevt2=Event disabled  dcaevt1src=DCAEVT1 with sync  dcaevt2src=DCAEVT2 with sync  dcbevt1src=DCBEVT1 with sync  dcbevt2src=DCBEVT2 with sync  pulsesel=Counter equals to zero (CTR=Zero)  blankinv=off  blankoffset=0  blankwidth=0  evsrcsel=Filtered version of DCAEVT1 (DCAEVT1FILT)  encape=off
  phase balancing (third harmonic injection)1 : Subsystem  Commented=on
  residue1 : Subsystem  Commented=on
  sorting1 : Subsystem  Commented=on
  ePWM_12 : Outport  VectorParamsAs1DForOutWhenUnconnected=off
  ePWM_11 : Outport  Port=2  VectorParamsAs1DForOutWhenUnconnected=off
  ePWM_10 : Outport  Port=3  VectorParamsAs1DForOutWhenUnconnected=off
  ePWM_6 : Outport  Port=4  VectorParamsAs1DForOutWhenUnconnected=off
  ePWM_5 : Outport  Port=5  VectorParamsAs1DForOutWhenUnconnected=off
  ePWM_4 : Outport  Port=6  VectorParamsAs1DForOutWhenUnconnected=off
  ePWM_3 : Outport  Port=7  VectorParamsAs1DForOutWhenUnconnected=off
  "ePWM_2 " : Outport  Port=8  VectorParamsAs1DForOutWhenUnconnected=off
  ePWM_1 : Outport  Port=9  VectorParamsAs1DForOutWhenUnconnected=off
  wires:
  Float to IQN5/1 -> Inverse Park Transformation/3
  Theta/1 -> Float to IQN5/1
  "u_d "/1 -> Float to IQN1/1
  Space Vector Generator/3 -> Mux/3
  Space Vector Generator/2 -> Mux/2
  Space Vector Generator/1 -> Mux/1
  10~90%/1 -> Shut_Off_PWM/1
  Inverse Park Transformation/1 -> Space Vector Generator/1
  Mux/1 -> Add/2
  Add/1 -> 10~90%/1
  Inverse Park Transformation/2 -> Space Vector Generator/2
  Constant7/1 -> Add/1
  "u_q "/1 -> Float to IQN2/1
  Constant1/1 -> Shut_Off_PWM/3
  On/Off/1 -> Shut_Off_PWM1/2, Shut_Off_PWM/2
  Shut_Off_PWM1/1 -> P123/1
  Constant2/1 -> Shut_Off_PWM1/3
  Constant3/1 -> Shut_Off_PWM1/1
  Float to IQN1/1 -> Inverse Park Transformation/1
  Float to IQN2/1 -> Inverse Park Transformation/2
  Demux4/1 -> ePWM_12/1
  Demux4/3 -> ePWM_10/1
  Demux4/2 -> ePWM_11/1
  Shut_Off_PWM/1 -> PWM_Scaling/1, PWM_Scaling1/1
  PWM_Scaling1/1 -> Demux4/1
  PWM_Scaling/1 -> Demux/1
  Constant5/1 -> sorting1/2(Ts)
  Data Store Read/1 -> Mux2/1
  PWM_Scaling2/1 -> Demux2/1
  Mux3/1 -> PWM_Scaling2/1
  Gain1/1 -> V-T conversion1/1
  Mux2/1 -> Gain1/1
  carier1/1(tr1) -> capacitor balancing1/3(Tri)
  capacitor balancing1/6(ePWM_1) -> Mux3/6
  Data Store Read3/1 -> Mux2/2
  Data Store Read4/1 -> Mux2/3
  capacitor balancing1/4(ePWM_3) -> Mux3/4
  capacitor balancing1/5(ePWM_2) -> Mux3/5
  capacitor balancing1/3(ePWM_4) -> Mux3/3
  sorting1/1(Tgabc) -> capacitor balancing1/2(Tabc)
  capacitor balancing1/1(ePWM_6) -> Mux3/1
  capacitor balancing1/2(ePWM_5) -> Mux3/2
  V-T conversion1/1 -> phase balancing (third harmonic injection)1/1(Tabc)
  phase balancing (third harmonic injection)1/1(Tabc_cross) -> capacitor balancing1/1(Tabc_cross), residue1/1(Tabc)
  residue1/1(Tabc_modified) -> sorting1/1(Tabc_cross)
  Demux/1 -> ePWM_5/1, ePWM_6/1
  Demux/2 -> ePWM_4/1, ePWM_3/1
  Demux/3 -> "ePWM_2 "/1, ePWM_1/1

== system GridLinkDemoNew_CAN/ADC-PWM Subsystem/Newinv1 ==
  note: Input: uint16 Output: sfix32_En16
  note: voltage amplified by 100: e.g., 12 V => 1200
  A4 : Inport  OutDataTypeStr=uint16  PortDimensions=1
  A5 : Inport  Port=2  OutDataTypeStr=uint16  PortDimensions=1
  A6 : Inport  Port=3  OutDataTypeStr=uint16  PortDimensions=1
  B0 : Inport  Port=4  OutDataTypeStr=uint16  PortDimensions=1
  B1 : Inport  Port=5  OutDataTypeStr=uint16  PortDimensions=1
  B2 : Inport  Port=6  OutDataTypeStr=uint16  PortDimensions=1
  theta : Inport  Port=7
  Current scaling + Clarke/Park : Subsystem
  Voltage scaling + Clarke/Park : Subsystem
  Vd : Outport  PortDimensions=1  VectorParamsAs1DForOutWhenUnconnected=off
  Vq : Outport  Port=2  PortDimensions=1  VectorParamsAs1DForOutWhenUnconnected=off
  Id : Outport  Port=3  PortDimensions=1  VectorParamsAs1DForOutWhenUnconnected=off
  Iq : Outport  Port=4  PortDimensions=1  VectorParamsAs1DForOutWhenUnconnected=off
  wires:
  A5/1 -> Voltage scaling + Clarke/Park/2(V_ADC_2)
  Voltage scaling + Clarke/Park/2(V_q (ADC)) -> Vq/1
  B0/1 -> Current scaling + Clarke/Park/1(I_ADC_1)
  A4/1 -> Voltage scaling + Clarke/Park/1(V_ADC_1)
  A6/1 -> Voltage scaling + Clarke/Park/3(V_ADC_3)
  B2/1 -> Current scaling + Clarke/Park/3(I_ADC_3)
  B1/1 -> Current scaling + Clarke/Park/2(I_ADC_2)
  [theta] -> Voltage scaling + Clarke/Park/4(Theta)
  [theta] -> Current scaling + Clarke/Park/4(Theta)
  theta/1 -> [theta]
  Current scaling + Clarke/Park/1(I_d (ADC)) -> Id/1
  Current scaling + Clarke/Park/2(I_q (ADC)) -> Iq/1
  Voltage scaling + Clarke/Park/1(V_d (ADC)) -> Vd/1

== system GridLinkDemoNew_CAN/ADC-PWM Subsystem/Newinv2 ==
  note: Input: uint16 Output: sfix32_En16
  note: voltage amplified by 100: e.g., 12 V => 1200
  A4 : Inport  OutDataTypeStr=uint16  PortDimensions=1
  A5 : Inport  Port=2  OutDataTypeStr=uint16  PortDimensions=1
  A6 : Inport  Port=3  OutDataTypeStr=uint16  PortDimensions=1
  B0 : Inport  Port=4  OutDataTypeStr=uint16  PortDimensions=1
  B1 : Inport  Port=5  OutDataTypeStr=uint16  PortDimensions=1
  B2 : Inport  Port=6  OutDataTypeStr=uint16  PortDimensions=1
  theta : Inport  Port=7
  Current scaling + Clarke/Park : Subsystem
  Voltage scaling + Clarke/Park : Subsystem
  Vd : Outport  PortDimensions=1  VectorParamsAs1DForOutWhenUnconnected=off
  Vq : Outport  Port=2  PortDimensions=1  VectorParamsAs1DForOutWhenUnconnected=off
  Id : Outport  Port=3  PortDimensions=1  VectorParamsAs1DForOutWhenUnconnected=off
  Iq : Outport  Port=4  PortDimensions=1  VectorParamsAs1DForOutWhenUnconnected=off
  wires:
  A5/1 -> Voltage scaling + Clarke/Park/2(V_ADC_2)
  Voltage scaling + Clarke/Park/2(V_q (ADC)) -> Vq/1
  B0/1 -> Current scaling + Clarke/Park/1(I_ADC_1)
  A4/1 -> Voltage scaling + Clarke/Park/1(V_ADC_1)
  A6/1 -> Voltage scaling + Clarke/Park/3(V_ADC_3)
  B2/1 -> Current scaling + Clarke/Park/3(I_ADC_3)
  B1/1 -> Current scaling + Clarke/Park/2(I_ADC_2)
  [theta] -> Voltage scaling + Clarke/Park/4(Theta)
  [theta] -> Current scaling + Clarke/Park/4(Theta)
  theta/1 -> [theta]
  Current scaling + Clarke/Park/1(I_d (ADC)) -> Id/1
  Current scaling + Clarke/Park/2(I_q (ADC)) -> Iq/1
  Voltage scaling + Clarke/Park/1(V_d (ADC)) -> Vd/1

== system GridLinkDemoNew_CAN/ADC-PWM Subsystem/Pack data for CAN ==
  In1 : Inport
  In2 : Inport  Port=2
  In3 : Inport  Port=3
  In4 : Inport  Port=4
  Byte Pack2 : svdutilitieslib/Byte Pack  maskPackedDataType=uint16  datatypes={'uint16' 'uint16' 'uint16' 'uint16'}  byteAlign=2  blockPlatform=tic2000
  Data Type Conversion7 : DataTypeConversion  OutDataTypeStr=uint16
  Demux4 : Demux
  Mux6 : Mux
  Output : Outport  OutDataTypeStr=uint16  VectorParamsAs1DForOutWhenUnconnected=off
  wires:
  Mux6/1 -> Data Type Conversion7/1
  In1/1 -> Mux6/1
  Data Type Conversion7/1 -> Demux4/1
  In2/1 -> Mux6/2
  In4/1 -> Mux6/4
  In3/1 -> Mux6/3
  Byte Pack2/1 -> Output/1
  Demux4/1 -> Byte Pack2/1
  Demux4/2 -> Byte Pack2/2
  Demux4/3 -> Byte Pack2/3
  Demux4/4 -> Byte Pack2/4

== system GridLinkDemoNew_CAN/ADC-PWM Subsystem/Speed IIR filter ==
  Speed : Inport
  Add : Sum  Inputs=+-
  Add1 : Sum
  Constant1 : Constant  OutDataTypeStr=fixdt(1,32,16)
  Constant2 : Constant  Value=.01  OutDataTypeStr=fixdt(1,32,16)
  Product : Product
  Product1 : Product
  Unit Delay : UnitDelay  SampleTime=-1  HasFrameUpgradeWarning=on
  Filtered speed : Outport  VectorParamsAs1DForOutWhenUnconnected=off
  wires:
  Product1/1 -> Add1/2
  Unit Delay/1 -> Product1/2
  Add/1 -> Product1/1
  Product/1 -> Add1/1
  Constant2/1 -> Add/2, Product/2
  Constant1/1 -> Add/1
  Add1/1 -> Filtered speed/1, Unit Delay/1
  Speed/1 -> Product/1

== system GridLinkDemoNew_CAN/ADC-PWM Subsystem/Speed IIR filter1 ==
  Speed : Inport
  Add : Sum  Inputs=+-
  Add1 : Sum
  Constant1 : Constant  OutDataTypeStr=fixdt(1,32,16)
  Constant2 : Constant  Value=.01  OutDataTypeStr=fixdt(1,32,16)
  Product : Product
  Product1 : Product
  Unit Delay : UnitDelay  SampleTime=-1  HasFrameUpgradeWarning=on
  Filtered speed : Outport  VectorParamsAs1DForOutWhenUnconnected=off
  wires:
  Product1/1 -> Add1/2
  Unit Delay/1 -> Product1/2
  Add/1 -> Product1/1
  Product/1 -> Add1/1
  Constant2/1 -> Add/2, Product/2
  Constant1/1 -> Add/1
  Add1/1 -> Filtered speed/1, Unit Delay/1
  Speed/1 -> Product/1

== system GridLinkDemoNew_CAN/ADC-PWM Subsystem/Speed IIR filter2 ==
  Speed : Inport
  Add : Sum  Inputs=+-
  Add1 : Sum
  Constant1 : Constant  OutDataTypeStr=fixdt(1,32,16)
  Constant2 : Constant  Value=.01  OutDataTypeStr=fixdt(1,32,16)
  Product : Product
  Product1 : Product
  Unit Delay : UnitDelay  SampleTime=-1  HasFrameUpgradeWarning=on
  Filtered speed : Outport  VectorParamsAs1DForOutWhenUnconnected=off
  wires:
  Product1/1 -> Add1/2
  Unit Delay/1 -> Product1/2
  Add/1 -> Product1/1
  Product/1 -> Add1/1
  Constant2/1 -> Add/2, Product/2
  Constant1/1 -> Add/1
  Add1/1 -> Filtered speed/1, Unit Delay/1
  Speed/1 -> Product/1

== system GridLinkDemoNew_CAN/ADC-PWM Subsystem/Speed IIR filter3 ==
  Speed : Inport
  Add : Sum  Inputs=+-
  Add1 : Sum
  Constant1 : Constant  OutDataTypeStr=fixdt(1,32,16)
  Constant2 : Constant  Value=.01  OutDataTypeStr=fixdt(1,32,16)
  Product : Product
  Product1 : Product
  Unit Delay : UnitDelay  SampleTime=-1  HasFrameUpgradeWarning=on
  Filtered speed : Outport  VectorParamsAs1DForOutWhenUnconnected=off
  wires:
  Product1/1 -> Add1/2
  Unit Delay/1 -> Product1/2
  Add/1 -> Product1/1
  Product/1 -> Add1/1
  Constant2/1 -> Add/2, Product/2
  Constant1/1 -> Add/1
  Add1/1 -> Filtered speed/1, Unit Delay/1
  Speed/1 -> Product/1

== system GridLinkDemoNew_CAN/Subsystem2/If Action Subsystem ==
  Action Port : ActionPort  ActionPortLabel=if(u1 >= u2)
  Constant : Constant  Value=0  OutDataTypeStr=single
  Data Store Write1 : DataStoreWrite  DataStoreName=Counter
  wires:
  Constant/1 -> Data Store Write1/1

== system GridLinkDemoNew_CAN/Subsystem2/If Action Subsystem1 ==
  Action Port : ActionPort  ActionPortLabel=else
  Data Store Read1 : DataStoreRead  DataStoreName=Counter
  Data Store Write1 : DataStoreWrite  DataStoreName=Counter
  Increment Stored Integer1 : simulink/Additional Math & Discrete/Additional Math: Increment - Decrement/Increment Stored Integer
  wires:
  Data Store Read1/1 -> Increment Stored Integer1/1
  Increment Stored Integer1/1 -> Data Store Write1/1

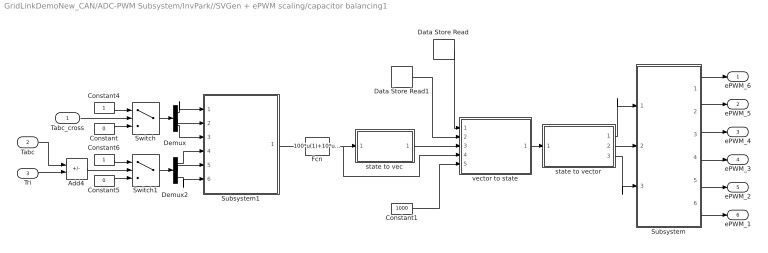
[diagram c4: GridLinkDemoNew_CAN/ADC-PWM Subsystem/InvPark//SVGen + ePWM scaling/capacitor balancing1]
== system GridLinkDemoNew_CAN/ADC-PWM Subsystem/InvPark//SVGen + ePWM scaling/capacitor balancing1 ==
  Tabc_cross : Inport
  Tabc : Inport  Port=2
  Tri : Inport  Port=3
  Add4 : Sum  Inputs=+-
  Constant : Constant  Value=0
  Constant1 : Constant  Value=1000
  Constant4 : Constant
  Constant5 : Constant  Value=0
  Constant6 : Constant
  Data Store Read : DataStoreRead  DataStoreName=VdcP
  Data Store Read1 : DataStoreRead  DataStoreName=VdcN
  Demux : Demux  Outputs=3
  Demux2 : Demux  Outputs=3
  Fcn : Fcn  Expr=100*u(1)+10*u(2)+u(3)
  Subsystem : Subsystem
  Subsystem1 : Subsystem
  Switch : Switch  Criteria=u2 > Threshold
  Switch1 : Switch  Criteria=u2 > Threshold
  state to vec : MATLAB Function  TreatAsAtomicUnit=on
  state to vector : MATLAB Function  TreatAsAtomicUnit=on
  vector to state : MATLAB Function  TreatAsAtomicUnit=on
  ePWM_6 : Outport  VectorParamsAs1DForOutWhenUnconnected=off
  ePWM_5 : Outport  Port=2  VectorParamsAs1DForOutWhenUnconnected=off
  ePWM_4 : Outport  Port=3  VectorParamsAs1DForOutWhenUnconnected=off
  ePWM_3 : Outport  Port=4  VectorParamsAs1DForOutWhenUnconnected=off
  ePWM_2 : Outport  Port=5  VectorParamsAs1DForOutWhenUnconnected=off
  ePWM_1 : Outport  Port=6  VectorParamsAs1DForOutWhenUnconnected=off
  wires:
  Constant1/1 -> vector to state/5(diff_V)
  Subsystem1/1(Ph_abc) -> Fcn/1
  Demux2/3 -> Subsystem1/6(PWM_c)
  Demux2/2 -> Subsystem1/5(PWM_b)
  Demux2/1 -> Subsystem1/4(PWM_a)
  Demux/3 -> Subsystem1/3(level_C)
  Demux/2 -> Subsystem1/2(level_B)
  Demux/1 -> Subsystem1/1(level_A)
  state to vec/1(Vector) -> vector to state/3(Vector)
  Switch1/1 -> Demux2/1
  Switch/1 -> Demux/1
  state to vector/3(c) -> Subsystem/3(c_ph_state)
  Tabc/1 -> Add4/1
  vector to state/1(state) -> state to vector/1(state)
  state to vector/2(b) -> Subsystem/2(b_ph_state)
  Tabc_cross/1 -> Switch/2
  state to vector/1(a) -> Subsystem/1(a_ph_state)
  Fcn/1 -> state to vec/1(state), vector to state/4(state1)
  Tri/1 -> Add4/2
  Add4/1 -> Switch1/2
  Constant5/1 -> Switch1/3
  Constant6/1 -> Switch1/1
  Constant/1 -> Switch/3
  Constant4/1 -> Switch/1
  Subsystem/1(ePWM_6) -> ePWM_6/1
  Subsystem/2(ePWM_5) -> ePWM_5/1
  Subsystem/3(ePWM_4) -> ePWM_4/1
  Subsystem/4(ePWM_3) -> ePWM_3/1
  Subsystem/5(ePWM_2) -> ePWM_2/1
  Subsystem/6(ePWM_1) -> ePWM_1/1
  Data Store Read/1 -> vector to state/1(Vc1)
  Data Store Read1/1 -> vector to state/2(Vc2)
